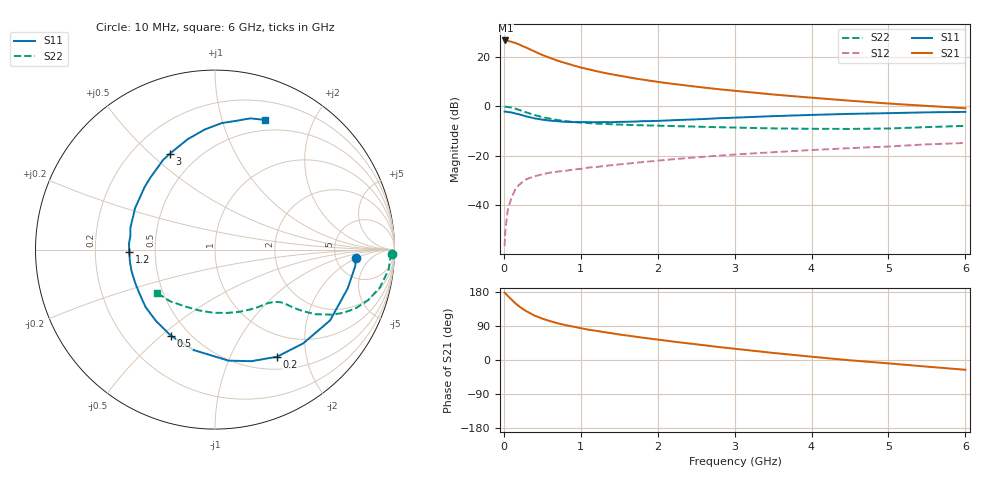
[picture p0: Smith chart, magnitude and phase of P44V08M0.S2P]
! SIEMENS Small Signal Semiconductors
! BFP182
! Si NPN RF Bipolar Junction Transistor in SOT143
! VCE = 4 V  IC = 8 mA
! Common Emitter S-Parameters:  March  1996
# GHz  S  MA  R  50
!  f  S11  S21  S12  S22
! GHz  MAG  ANG  MAG  ANG  MAG  ANG  MAG  ANG
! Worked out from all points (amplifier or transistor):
!   36 points, 10 MHz to 6 GHz, reference 50 ohm
!   highest |S21| = 26.6 dB at 20 MHz (marker M1)
!   |S21| within 3 dB of that: start of sweep to 299.7 MHz
!   unconditionally stable (mu >= 1): 1.329 GHz to 5.404 GHz
!   at 250 MHz: K = 0.28, MSG = 27.3 dB, |S12| = -30.4 dB
!   at 1.4 GHz: K = 1.03, MAG = 17.3 dB, |S12| = -23.8 dB
!   at 6 GHz: K = 0.95, MSG = 7.0 dB, |S12| = -14.8 dB
!   lowest NFmin = 1.40 dB at 450 MHz
!   S11 on the Smith chart (normalised r, x): 10 MHz: 7.85, -1.84; 200 MHz: 0.67, -1.52; 500 MHz: 0.40, -0.54; 1.2 GHz: 0.35, -0.01; 3 GHz: 0.35, +0.58; 6 GHz: 0.38, +1.38
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0.01  0.7846 -3.3  21.15 177.8  0.0015 79.1  0.985 -1.3
0.02  0.787 -6.6  21.44 176.0  0.0031 86.1  0.9785 -2.6
0.05  0.7703 -16.3  21.13 169.3  0.0079 84.0  0.9737 -6.6
0.1  0.7529 -31.6  20.09 159.3  0.0145 73.9  0.9435 -12.8
0.15  0.7172 -46.8  19.1 149.7  0.0212 67.2  0.899 -18.3
0.2  0.6895 -60.0  17.79 141.4  0.0262 62.5  0.8476 -22.8
0.25  0.6538 -72.0  16.32 134.2  0.0303 57.0  0.7974 -26.2
0.3  0.6231 -83.1  15.17 128.0  0.0341 53.5  0.748 -29.0
0.4  0.5722 -101.9  12.83 117.1  0.0387 48.1  0.6665 -32.7
0.5  0.5394 -117.0  10.91 109.2  0.0425 44.6  0.6068 -34.7
0.6  0.5158 -129.6  9.547 102.6  0.0458 42.6  0.5632 -36.0
0.7  0.502 -140.5  8.351 97.0  0.0481 42.2  0.5293 -36.8
0.9  0.4819 -157.5  6.746 88.1  0.0529 40.9  0.4844 -38.0
1.1  0.4787 -172.3  5.612 80.1  0.058 41.0  0.459 -39.5
1.2  0.4777 -178.2  5.155 77.0  0.0595 40.7  0.4497 -40.4
1.7  0.4931 157.1  3.676 61.9  0.0721 41.5  0.4181 -45.7
2.2  0.525 138.3  2.844 48.6  0.0853 40.4  0.4005 -53.1
3  0.5912 115.1  2.066 29.7  0.1064 36.4  0.373 -68.2
3.5  0.6344 103.7  1.738 18.7  0.1186 33.3  0.3591 -79.3
4.5  0.7056 87.0  1.301 -0.8  0.1432 26.6  0.3503 -104.8
5.5  0.7573 74.9  1.022 -17.5  0.171 19.8  0.3812 -131.0
6  0.7738 69.1  0.917 -25.8  0.1823 15.2  0.4044 -143.5
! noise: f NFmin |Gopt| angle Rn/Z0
0.45  1.4  0.26  41  0.29
0.9  1.5  0.25  83  0.23
1.8  2  0.21  162  0.2
